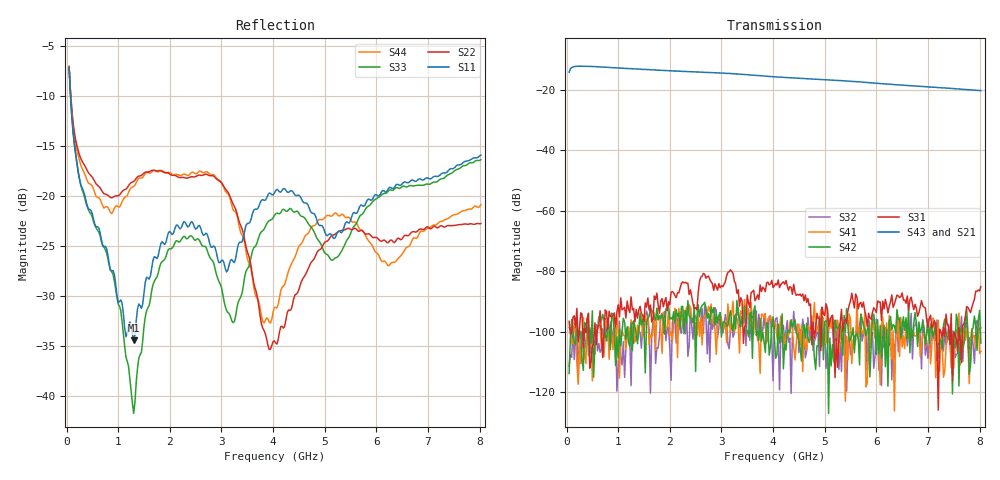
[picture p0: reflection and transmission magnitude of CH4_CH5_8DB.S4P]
!Agilent Technologies,E5071C,MY46316741,A.11.02
!Date: Mon Jun 01 11:47:34 2026
!Data & Calibration Information:
!1:CH4 INPUT 2:CH4 OUTPUT 3:CH5 INPUT 4:CH5 OUTPUT
!Freq	S11:SOLT4(ON)	S12:SOLT4(ON)	S13:SOLT4(ON)	S14:SOLT4(ON)
!	S21:SOLT4(ON)	S22:SOLT4(ON)	S23:SOLT4(ON)	S24:SOLT4(ON)
!	S31:SOLT4(ON)	S32:SOLT4(ON)	S33:SOLT4(ON)	S34:SOLT4(ON)
!	S41:SOLT4(ON)	S42:SOLT4(ON)	S43:SOLT4(ON)	S44:SOLT4(ON)
!PortZ  Port1:50+j0  Port2:50+j0  Port3:50+j0  Port4:50+j0
!Above PortZ is port z conversion or system Z0 setting when saving the data.
!When reading, reference impedance value at option line is always used.
# Hz S dB R 50
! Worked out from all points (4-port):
!   320 points, 50 MHz to 8.025 GHz, reference 50 ohm
!   strongest paths, dB at 50 MHz, 2.05 GHz, 4.05 GHz, 6.05 GHz, 8.025 GHz:
!     S43: -14.2, -13.7, -15.7, -17.9, -20.3
!     S21: -14.2, -13.8, -15.9, -18.0, -20.4
!     S31: -96.6, -86.7, -84.1, -90.2, -85.1
!     S42: -113.8, -95.9, -108.8, -107.3, -103.8
!     S41: -98.6, -103.2, -97.5, -105.7, -106.5
!     S32: -111.4, -97.2, -95.8, -112.7, -98.7
!   lowest |S11| = -34.4 dB at 1.3 GHz (marker M1), VSWR 1.04, Z = 48.5 - j1.16 ohm
!   |S11| at or under -10 dB: 77.03 MHz to end of sweep
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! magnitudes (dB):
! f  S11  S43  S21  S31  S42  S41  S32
! 50 MHz  -7.2  -14.2  -14.2  -96.6  -113.8  -98.6  -111.4
! 425 MHz  -21.3  -12.2  -12.3  -93.9  -107.9  -102.9  -95.9
! 1.3 GHz  -34.4  -13.1  -13.2  -92.4  -96.4  -96.8  -103.9
! 1.975 GHz  -23.7  -13.7  -13.8  -90.2  -91.4  -93.0  -98.5
! 3.225 GHz  -26.6  -14.7  -14.8  -80.7  -100.0  -90.0  -101.8
! 3.925 GHz  -19.7  -15.6  -15.8  -84.5  -107.8  -95.7  -94.9
! 8.025 GHz  -15.9  -20.3  -20.4  -85.1  -103.8  -106.5  -98.7
